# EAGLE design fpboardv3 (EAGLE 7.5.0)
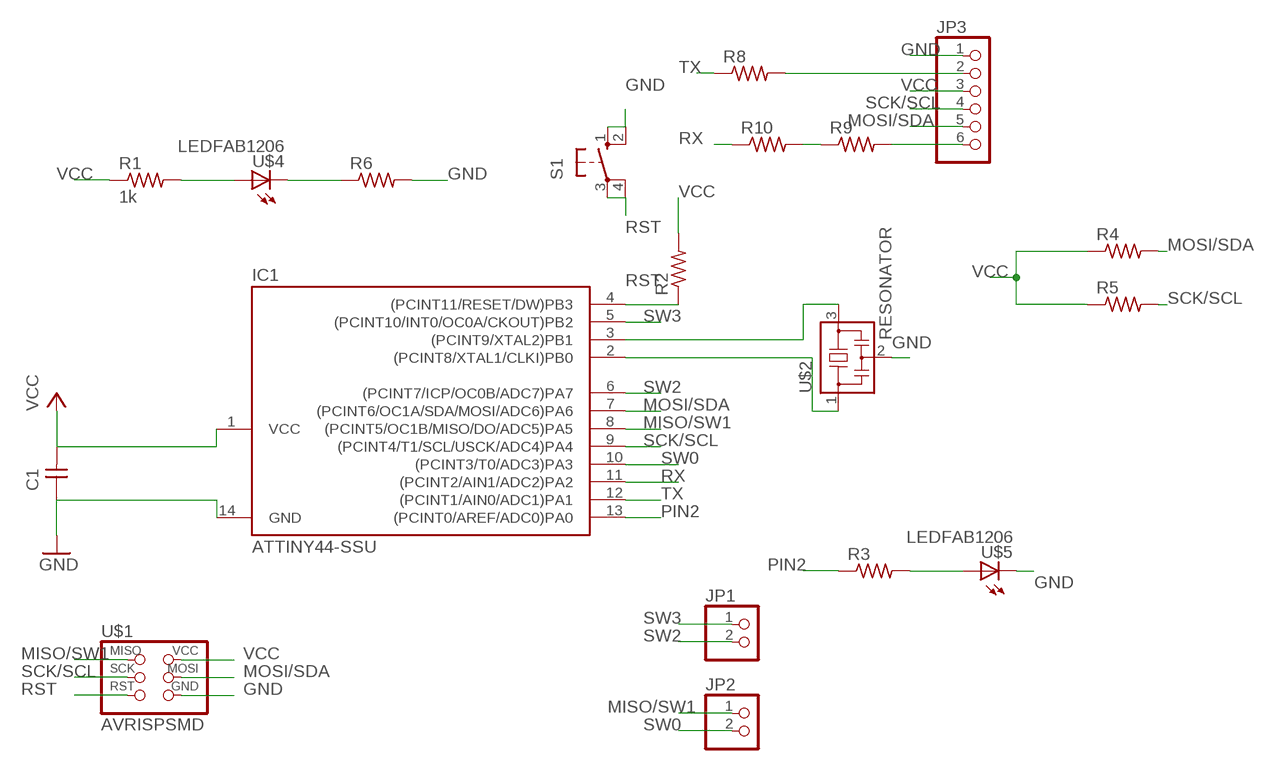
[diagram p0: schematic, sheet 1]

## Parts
C1  CAP-UNPOLARIZEDFAB  [C1206FAB]
IC1  ATTINY44-SSU  [SOIC14]
JP1  PINHD-1X2  [1X02]
JP2  PINHD-1X2  [1X02]
JP3  PINHD-1X6  [1X06]
R1  1k  RES-US1206FAB  [R1206FAB]
R2  RES-US1206FAB  [R1206FAB]
R3  RES-US1206FAB  [R1206FAB]
R4  RES-US1206FAB  [R1206FAB]
R5  RES-US1206FAB  [R1206FAB]
R6  RES-US1206FAB  [R1206FAB]
R8  RES-US1206FAB  [R1206FAB]
R9  RES-US1206FAB  [R1206FAB]
R10  RES-US1206FAB  [R1206FAB]
S1  10-XX  [B3F-10XX]
U$1  AVRISPSMD  [2X03SMD]
U$2  RESONATOR  [EFOBM]
U$4  LEDFAB1206  [LED1206FAB]
U$5  LEDFAB1206  [LED1206FAB]

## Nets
GND: C1.1 IC1.14(GND) JP3.1 R6.1 R6.2 S1.1(S) S1.2(S1) U$1.6(GND) U$2.2 U$4.2(C) U$5.2(C)
MISO/SW1: IC1.8((PCINT5/OC1B/MISO/DO/ADC5)PA5) JP2.1 U$1.1(MISO)
MOSI/SDA: IC1.7((PCINT6/OC1A/SDA/MOSI/ADC6)PA6) JP3.5 R4.2 U$1.4(MOSI)
N$1: IC1.2((PCINT8/XTAL1/CLKI)PB0) U$2.1
N$2: IC1.3((PCINT9/XTAL2)PB1) U$2.3
N$3: R1.2 U$4.1(A)
N$4: R3.2 U$5.1(A)
N$5: R9.1 R10.2
N$8: JP3.2 R8.2
N$9: JP3.6 R9.2
PIN2: IC1.13((PCINT0/AREF/ADC0)PA0) R3.1
RST: IC1.4((PCINT11/RESET/DW)PB3) R2.1 S1.3(P) S1.4(P1) U$1.5(RST)
RX: IC1.11((PCINT2/AIN1/ADC2)PA2) R10.1
SCK/SCL: IC1.9((PCINT4/T1/SCL/USCK/ADC4)PA4) JP3.4 R5.2 U$1.3(SCK)
SW0: IC1.10((PCINT3/T0/ADC3)PA3) JP2.2
SW2: IC1.6((PCINT7/ICP/OC0B/ADC7)PA7) JP1.2
SW3: IC1.5((PCINT10/INT0/OC0A/CKOUT)PB2) JP1.1
TX: IC1.12((PCINT1/AIN0/ADC1)PA1) R8.1
VCC: C1.2 IC1.1(VCC) JP3.3 R1.1 R2.2 R4.1 R5.1 U$1.2(VCC)

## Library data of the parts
C1 = fab:CAP-UNPOLARIZED
IC1 = fab:ATTINY44
JP1 JP2 = pinhead:PINHD-1X2: PIN HEADER
JP3 = pinhead:PINHD-1X6: PIN HEADER
R1-R6 R8-R10 = fab:RES-US: Resistor (US Symbol)
S1 = switch-omron:10-XX: OMRON SWITCH; MPN: B3F-1000; OC_FARNELL: 176432; OC_NEWARK: 36M3542
U$1 = fab:AVRISP
U$2 = fab:RESONATOR
U$4 U$5 = fab:LED: LED

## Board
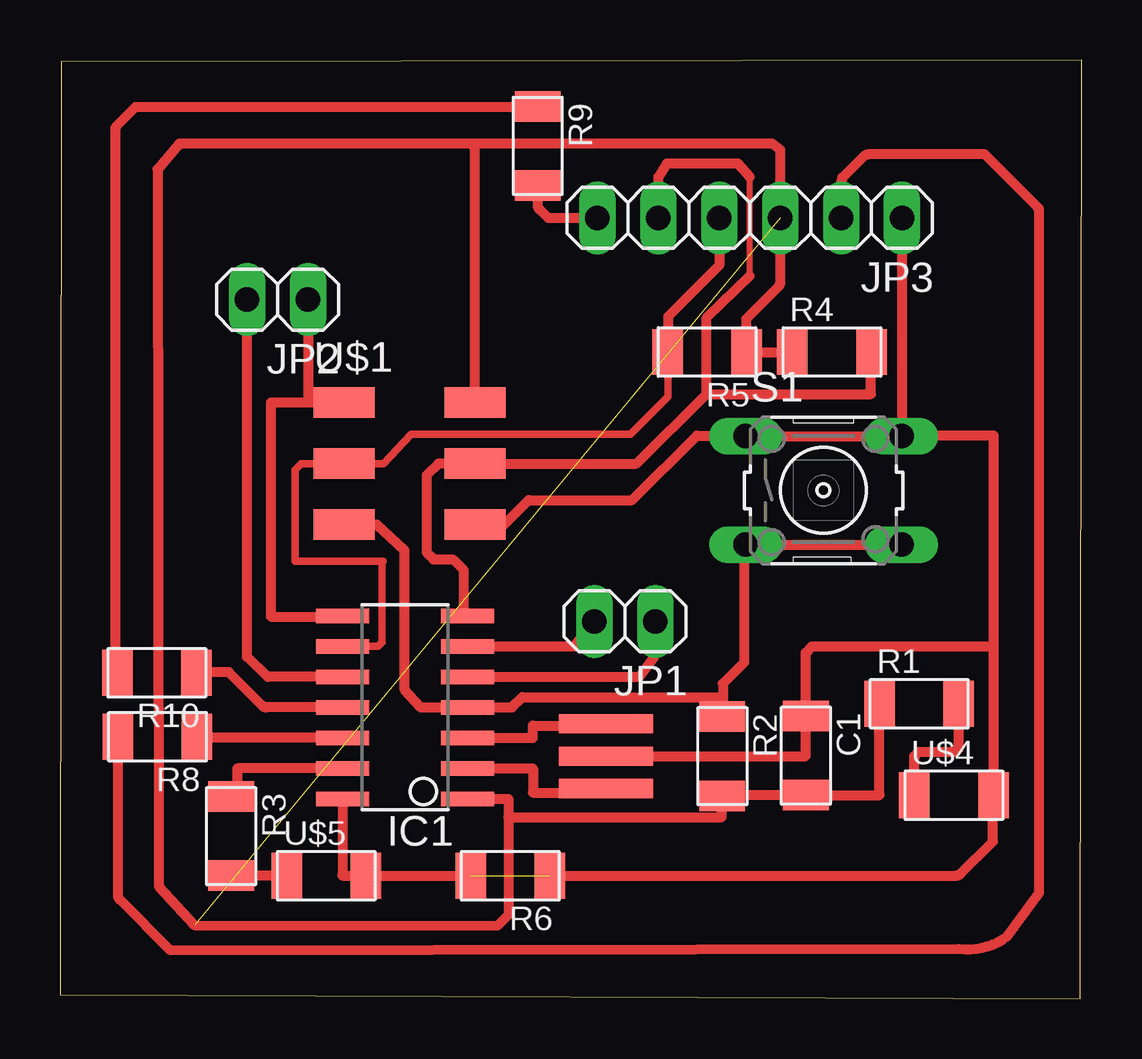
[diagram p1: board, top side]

Size 42.6 x 39.12 mm. Coordinates in mm from the lower left corner, seen from the top.
Outline: 0,0.18 42.53,0 42.6,39.12 0.05,39.04 0,0.18
Copper layers (1*16): Top 0.035mm / dielectric 1.5mm / Bottom 0.035mm
Design rules "default *": minimum track width 10mil, minimum drill 24mil, track to track 15mil, track to pad 15mil, pad to pad 15mil, via to via 15mil, smd to smd 15mil, copper to edge 40mil, drill to drill 8mil, minimum pad ring 10mil, minimum via ring 8mil, stop-mask expansion 4mil, vias tented up to drill 0mil, thermal gap 10mil

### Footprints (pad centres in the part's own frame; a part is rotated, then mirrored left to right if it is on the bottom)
C1206FAB = smd 1.27 x 1.905: 1 -1.651,0; 2 1.651,0
SOIC14 = smd 0.61 x 2.21: 1 -3.81,-2.603; 2 -2.54,-2.603; 3 -1.27,-2.603; 4 0,-2.603; 5 1.27,-2.603; 6 2.54,-2.603; 7 3.81,-2.603; 8 3.81,2.603; 9 2.54,2.603; 10 1.27,2.603; 11 0,2.603; 12 -1.27,2.603; 13 -2.54,2.603; 14 -3.81,2.603
1X02 = drill 1.016 long: 1 -1.27,0; 2 1.27,0
1X06 = drill 1.016 long: 1 -6.35,0; 2 -3.81,0; 3 -1.27,0; 4 1.27,0; 5 3.81,0; 6 6.35,0
R1206FAB = smd 1.27 x 1.905: 1 -1.651,0; 2 1.651,0
B3F-10XX = drill 1.016 long: 1 -3.251,2.261; 2 3.251,2.261; 3 -3.251,-2.261; 4 3.251,-2.261
2X03SMD = smd 2.54 x 1.27: 1 -2.54,2.54; 2 2.92,2.54; 3 -2.54,0; 4 2.92,0; 5 -2.54,-2.54; 6 2.92,-2.54
EFOBM = smd 0.8 x 3.9: 1 -1.35,0; 2 0,0; 3 1.35,0
LED1206FAB = smd 1.27 x 1.905: 1 -1.651,0; 2 1.651,0

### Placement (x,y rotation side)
C1  31.09,10.13 270 top
IC1  14.38,12.14 90 top
JP1  23.55,15.72 180 top
JP2  9.07,29.13 180 top
JP3  28.75,32.54 180 top
R1  35.81,12.29 0 top
R2  27.61,10.11 270 top
R3  7.14,6.78 270 top
R4  32.18,26.95 0 top
R5  26.97,26.95 180 top
R6  18.77,5.13 180 top
R8  4.06,10.92 180 top
R9  19.91,35.53 270 top
R10  4.04,13.59 180 top
S1  31.83,21.18 0 top
U$1  14.38,22.3 0 top
U$2  22.76,10.11 90 top
U$4  37.26,8.48 0 top
U$5  11.1,5.13 0 top

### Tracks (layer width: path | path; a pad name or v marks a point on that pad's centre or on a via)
GND  (1 unrouted)
  Top 0.406: U$2.2 31.09,10.11 C1.1 31.09,14.43 31.34,14.68 38.91,14.68 | 38.91,14.68 38.91,23.47 35.14,23.47 arc45 S1.2 | 38.91,14.68 U$4.2 arc45 38.89,8.42 38.89,6.55 37.54,5.21 arc-45 37.36,5.13 R6.1 | U$1.6 18.52,19.76 19.53,20.78 23.85,20.78 26.54,23.47 28.51,23.47 arc-45 S1.1 S1.2 | IC1.14 11.77,5.16 arc45 11.79,5.13 U$5.2 R6.2 | 35.1,23.51 arc-45 S1.2 | JP3.1 35.1,23.47
  Top 0.61: 35.1,23.47 S1.2
MISO/SW1
  Top 0.406: U$1.1 10.49,24.84 | 10.49,24.84 8.79,24.84 8.79,15.93 11.77,15.93 IC1.8 | JP2.1 10.34,24.99 10.49,24.84
MOSI/SDA
  Top 0.254: 28.75,30.12 28.75,34.24
  Top 0.406: IC1.7 16.81,16.12 16.81,17.88 16.38,18.31 15.57,18.31 15.29,18.59 15.29,21.82 15.77,22.3 U$1.4 24.03,22.3 26.95,25.2 | 26.95,25.2 26.95,28.37 28.75,30.12 | 28.75,34.24 28.27,34.8 25.3,34.8 24.94,34.24 JP3.5 | 26.95,25.2 33.81,25.2 R4.2
N$1
  Top 0.406: IC1.2 19.71,9.6 19.71,8.59 22.76,8.59 U$2.1
N$2
  Top 0.406: IC1.3 19.71,10.87 19.71,11.38 22.76,11.38 U$2.3
N$3
  Top 0.406: U$4.1 35.61,10.11 35.79,10.29 37.34,10.29 37.47,10.41 R1.2
N$4
  Top 0.406: U$5.1 R3.2
N$5
  Top 0.406: R10.2 2.39,13.61 arc45 2.31,13.79 2.31,36.22 arc-45 2.39,36.4 3.15,37.16 19.85,37.16 arc45 R9.1
N$8
  Top 0.406: R8.2 2.41,4.32 arc45 2.49,4.14 4.6,2.03 37.49,2.08 arc45 39.5,2.61 40.82,4.42 40.82,32.81 arc45 40.74,32.99 38.56,35.18 33.68,35.18 arc45 33.5,35.1 32.61,34.21 32.61,34.18 arc-45 32.56,34.06 JP3.2
N$9
  Top 0.406: R9.2 19.91,33.07 arc45 19.99,32.9 20.35,32.54 JP3.6
PIN2
  Top 0.406: IC1.13 7.45,9.6 arc45 7.39,9.58 7.39,8.79 arc-45 7.32,8.61 R3.1
RST
  Top 0.406: 28.22,12.14 R2.1 27.64,11.79 27.64,12.65 | U$1.5 13.21,19.76 14.35,18.69 14.35,12.9 15.04,12.14 IC1.4 18.85,12.14 19.28,12.57 27.56,12.57 27.64,12.65 | 27.64,12.65 27.64,13.13 28.52,14.02 28.52,18.8 arc-45 S1.3 S1.4
RX
  Top 0.406: IC1.11 8.61,12.14 arc-45 8.43,12.22 7.04,13.61 5.75,13.61 arc45 R10.1
SCK/SCL
  Top 0.305: IC1.9 13.26,14.68 13.44,14.86 13.44,18.21 13.46,18.24 9.8,18.24 9.8,22.05 10.06,22.3 U$1.3 13.49,22.3 14.63,23.52 23.77,23.52 25.35,25.1 25.35,27.48
  Top 0.406: R5.2 25.35,27.48 25.35,28.42 27.48,30.56 JP3.4
SW0
  Top 0.406: IC1.10 8.66,13.41 7.8,14.25 JP2.2
SW2
  Top 0.406: IC1.6 21.44,14.68 JP1.2
SW3
  Top 0.406: IC1.5 24.16,13.41 24.74,14.2 JP1.1
TX
  Top 0.406: IC1.12 5.84,10.87 arc-45 R8.1
VCC  (1 unrouted)
  Top 0.254: 30.86,8.51 C1.2 | 27.79,8.51 R2.2
  Top 0.406: IC1.1 18.69,8.33 18.69,7.57 | 18.69,7.57 27.58,7.57 27.58,8.43 R2.2 | R1.1 34.16,8.48 C1.2 31.06,8.51 27.79,8.51 | 17.15,35.64 29.69,35.64 30.02,35.38 30.02,29.85 arc-45 29.95,29.67 28.6,28.32 28.6,27.01 arc45 R5.1 R4.1 | 17.15,35.64 4.98,35.64 4.06,34.57 4.11,4.7 5.61,3.07 18.24,3.05 18.72,3.53 18.72,7.54 18.69,7.57 | U$1.2 17.3,35.49 17.15,35.64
